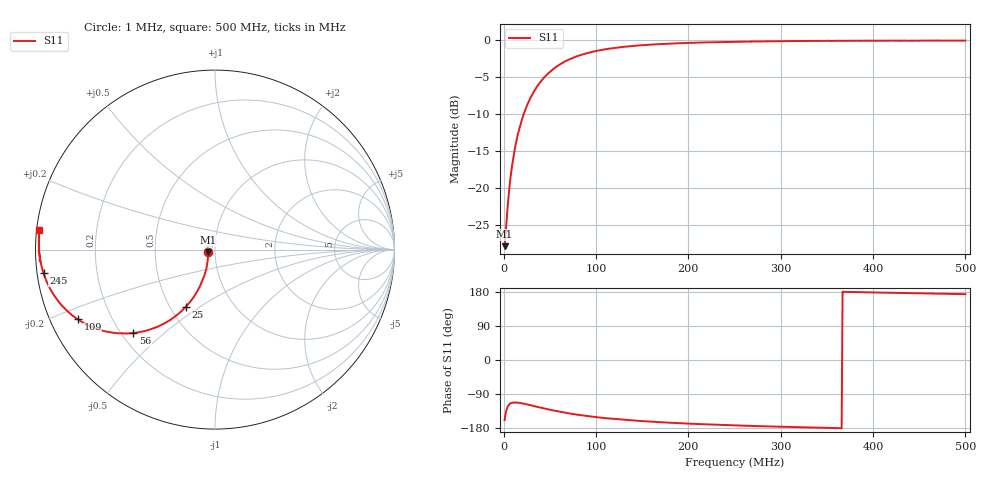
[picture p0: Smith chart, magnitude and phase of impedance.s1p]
# Hz S RI R 50.0
! written by SimSmith version 18.3b
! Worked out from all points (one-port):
!   500 points, 1 MHz to 500 MHz, reference 50 ohm
!   lowest |S11| = -27.8 dB at 1 MHz (marker M1), VSWR 1.08, Z = 46.3 - j1.37 ohm
!   |S11| at or under -10 dB: start of sweep to 21.8 MHz
!   S11 on the Smith chart (normalised r, x): 1 MHz: 0.93, -0.03; 25 MHz: 0.60, -0.44; 56 MHz: 0.25, -0.40; 109 MHz: 0.08, -0.24; 245 MHz: 0.02, -0.07; 500 MHz: 0.01, +0.05
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1000000  -0.0379 -0.0148
2000000  -0.0383 -0.0295
3000000  -0.0395 -0.0438
5000000  -0.0428 -0.0726
7000000  -0.0472 -0.1026
9000000  -0.0551 -0.1291
1.1e7  -0.0638 -0.1558
1.4e7  -0.0799 -0.1948
1.7e7  -0.0988 -0.2328
2.1e7  -0.1282 -0.2775
2.5e7  -0.1616 -0.3181
3.1e7  -0.2172 -0.3682
3.9e7  -0.2943 -0.4175
4.7e7  -0.3721 -0.4483
5.6e7  -0.4543 -0.4648
6.4e7  -0.5189 -0.4653
8.4e7  -0.6525 -0.4435
9.8e7  -0.7212 -0.4141
1.09e8  -0.7646 -0.3884
1.26e8  -0.8168 -0.348
1.55e8  -0.8761 -0.2836
1.89e8  -0.9183 -0.2184
2.45e8  -0.9553 -0.1317
2.51e8  -0.9578 -0.1235
3.13e8  -0.9755 -0.0517
3.76e8  -0.9806 0.00893
4.38e8  -0.9794 0.0597
5e8  -0.978 0.1071
